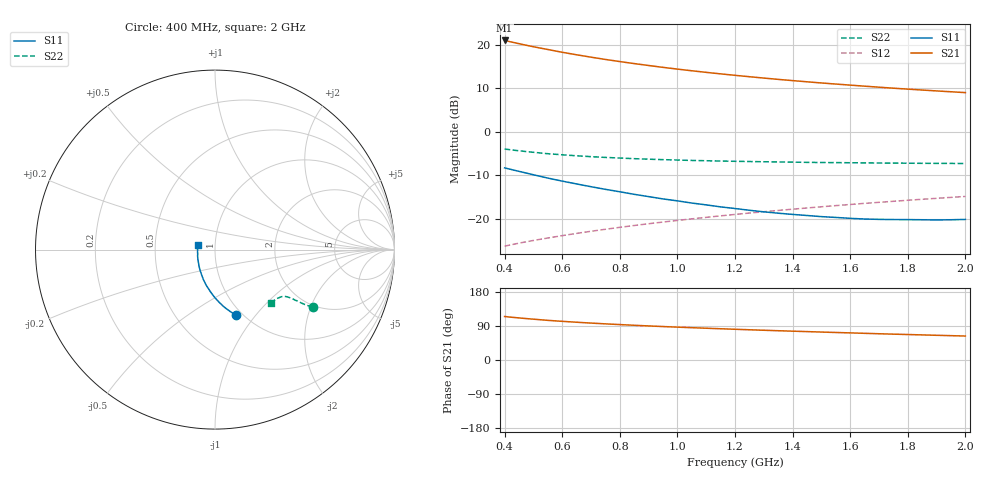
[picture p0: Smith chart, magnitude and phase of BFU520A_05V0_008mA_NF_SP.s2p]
! Filename:  P:\Prog\Test\Noise\ATS_data\Testdata_Net\06 Compressed Noise after Statistics\BFU520A_APG2013_30_A05_05p0V_008mA_NF_CM01_D.sf
! Date/Time: Wed 24/Apr/2013 20:06:18
! BFU520A_APG2013_30_A05_05p0V_1to20mA_NF_CM01_Bias5_R.sf
! Noise Parameter Data File
! BFU520A_APG2013_30_A05_05p0V_1to20mA_NF_CM01
! Date/time: Thu Apr 11 01:07:08 2013
! VAR V_out= 5.001000
! VAR I_out= 7.995000
! VAR V_in= 0.838000
! VAR I_in= 0.088310
! Device data file deembeded for feedlines and parallel
! Original file: \06 Compressed Noise after Statistics\BFU520A_APG2013_30_A05_05p0V_008mA_NF_CM01_R.sf
! Feed-files: PR017V01_150413_Feed1.s2p, PR017V01_150413_Feed2.s2p
! Parallel-file: PR017V01_150413_Par.s2p
# MHz S MA R 50
!  Freq-MHz  S11-mag  S11-arg  S21-mag  S21-arg  S12-mag  S12-arg  S22-mag  S22-arg
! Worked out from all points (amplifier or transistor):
!   37 points, 400 MHz to 2 GHz, reference 50 ohm
!   highest |S21| = 21.0 dB at 400 MHz (marker M1)
!   |S21| within 3 dB of that: start of sweep to 624.2 MHz
!   unconditionally stable (mu >= 1): 1.382 GHz to end of sweep
!   at 500 MHz: K = 0.77, MSG = 22.3 dB, |S12| = -25.0 dB
!   at 1.1 GHz: K = 0.98, MSG = 16.7 dB, |S12| = -19.7 dB
!   at 2 GHz: K = 1.01, MAG = 11.4 dB, |S12| = -14.9 dB
!   lowest NFmin = 0.77 dB at 420 MHz
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400  0.3835 -72.1  11.22 114.8  0.04817 66.9  0.6317 -30.5
420  0.3696 -74.1  10.83 113.2  0.04978 66.9  0.6195 -30.8
440  0.3558 -76.1  10.48 111.7  0.05136 66.8  0.6085 -31.0
460  0.3434 -77.9  10.13 110.3  0.05294 66.9  0.5984 -31.2
480  0.3315 -79.8  9.804 109.0  0.05448 66.9  0.5882 -31.4
500  0.3197 -81.6  9.499 107.7  0.05604 66.9  0.5796 -31.6
550  0.2925 -85.8  8.828 104.6  0.05978 67.1  0.5583 -31.8
600  0.2701 -89.7  8.204 102.0  0.06367 67.4  0.5422 -31.9
650  0.2505 -93.3  7.674 99.7  0.06756 67.6  0.5282 -32.2
700  0.2328 -96.9  7.205 97.4  0.07145 67.9  0.5163 -32.3
750  0.2172 -100.4  6.783 95.4  0.07537 68.2  0.5059 -32.5
800  0.2036 -104.1  6.413 93.5  0.07933 68.4  0.4974 -32.7
850  0.1903 -107.5  6.08 91.6  0.08328 68.5  0.4896 -32.9
950  0.1685 -114.4  5.501 88.3  0.09128 68.9  0.477 -33.4
1050  0.151 -121.2  5.025 85.3  0.0993 69.1  0.467 -33.9
1150  0.1364 -128.8  4.629 82.5  0.1075 69.2  0.4593 -34.6
1200  0.1307 -132.2  4.454 81.1  0.1117 69.3  0.4563 -35.0
1350  0.1154 -143.7  4.001 77.2  0.1242 69.2  0.4488 -36.3
1500  0.1054 -156.0  3.638 73.8  0.1368 69.0  0.442 -37.8
1650  0.0989 -167.7  3.342 70.4  0.1497 68.6  0.438 -39.6
1750  0.09751 -175.8  3.168 68.2  0.1582 68.3  0.4351 -40.7
2000  0.09778 166.5  2.817 63.2  0.1799 67.3  0.4304 -44.0
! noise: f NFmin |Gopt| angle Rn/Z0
400  0.8171  0.05101  7.15  0.1078
460  0.7875  0.04874  37.19  0.1027
600  0.8982  0.06353  13.28  0.1294
800  0.8355  0.01382  86.9  0.1017
1000  0.8617  0.03346  116.5  0.0975
1200  0.9104  0.03782  147  0.0985
1400  0.9473  0.05179  158.3  0.0959
1600  0.9486  0.07547  -166.1  0.0915
1800  0.9478  0.1164  -157.4  0.0845
2000  0.9003  0.1306  -129.5  0.1066
